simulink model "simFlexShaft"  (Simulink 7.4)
settings: Solver=ode45  StartTime=0.0  StopTime=inf  RelTol=1e-3
InitFcn:
  | updateVarParamFlexShaft
StopFcn:
  | stopFcnFlexShaft
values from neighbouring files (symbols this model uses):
  cmd = 0    [initFcnFlexShaft.m]    (also in updateVarParamFlexShaft.m = 1)
  controllerSel = 0    [initFcnFlexShaft.m]    (also in updateVarParamFlexShaft.m)
  denzTfLoopShapingController = [1 1e-3*ones(1,3)]    [initFcnFlexShaft.m]    (also in updateVarParamFlexShaft.m = Grd.den{1,1})
  fcnSel = 0    [initFcnFlexShaft.m]    (also in updateVarParamFlexShaft.m = 2)
  feedbackGainObserver = 1e-3*ones(N,1)    [initFcnFlexShaft.m]    (also in updateVarParamFlexShaft.m = L)
  feedbackGainStateController = 1e-3*ones(1,N)    [initFcnFlexShaft.m]    (also in updateVarParamFlexShaft.m = K_bar(1,2:end))
  integralGainPidController = 0.0    (= 0)    [initFcnFlexShaft.m]    (also in updateVarParamFlexShaft.m)
  integralGainStateController = 0.0    (= 0)    [initFcnFlexShaft.m]    (also in updateVarParamFlexShaft.m = K_bar(1,1))
  numzTfLoopShapingController = 1e-3*ones(1,4)    [initFcnFlexShaft.m]    (also in updateVarParamFlexShaft.m = Grd.num{1,1})
  proportionalGainPidController = 0.0    (= 0)    [initFcnFlexShaft.m]    (also in updateVarParamFlexShaft.m)
  sysMatrixAcPlant = sysc.Ac    [initFcnFlexShaft.m]    (also in updateVarParamFlexShaft.m)
  sysMatrixAdObserver = sysd.a    [initFcnFlexShaft.m]    (also in updateVarParamFlexShaft.m = Ad)
  sysMatrixBcPlant = sysc.Bc    [initFcnFlexShaft.m]    (also in updateVarParamFlexShaft.m)
  sysMatrixBduObserver = sysd.b(:,1)    [initFcnFlexShaft.m]    (also in updateVarParamFlexShaft.m = Bd(:,1))
  sysMatrixCcPlant = sysc.Cc    [initFcnFlexShaft.m]    (also in updateVarParamFlexShaft.m)
  sysMatrixCdObserver = sysd.c    [initFcnFlexShaft.m]    (also in updateVarParamFlexShaft.m = Cd)
  sysMatrixDcPlant = sysc.Dc    [initFcnFlexShaft.m]    (also in updateVarParamFlexShaft.m)
undefined symbols (not defined in the file or in its folder): constParamFlexShaft
libraries: simulink x14, dspsnks4 x2, simulink_extras x1
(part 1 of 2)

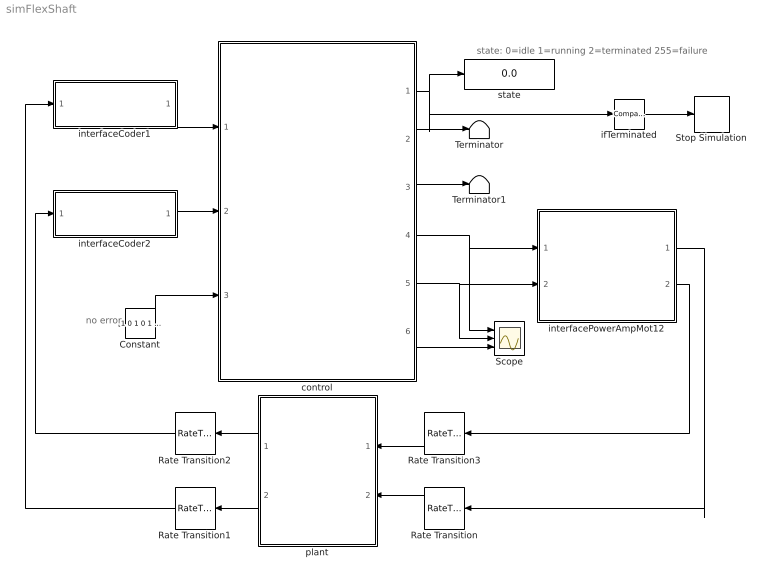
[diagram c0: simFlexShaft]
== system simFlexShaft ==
  note: state: 0=idle 1=running 2=terminated 255=failure
  note: no error
  Constant : Constant  Value=[1 0 1 0 1 0 0 0 0 0 0 0]
  Rate Transition{,1..3} (4 alike) : RateTransition
  Scope : Scope  NumInputPorts=3
  Stop Simulation : Stop
  Terminator : Terminator
  Terminator1 : Terminator
  control : Subsystem  TreatAsAtomicUnit=on  SystemSampleTime=constParamFlexShaft.samplingTime  mask{constParam=constParamFlexShaft.control, cmd=cmd, fcnSel=fcnSel, controllerSel=controllerSel, proportionalGainPidController=proportionalGainPidController, integralGainPidController=integralGainPidController, numzTfLoopShapingController=numzTfLoopShapingController, denzTfLoopShapingController=denzTfLoopShapingController, integralGainStateController=integralGainStateController, feedbackGainStateController=feedbackGainStateController, sysMatrixAdObserver=sysMatrixAdObserver, sysMatrixBduObserver=sysMatrixBduObserver, sysMatrixCdObserver=sysMatrixCdObserver, feedbackGainObserver=feedbackGainObserver}
      mask prompts: constParam "Constant:"; cmd "Command:"; fcnSel "Function Selector:"; controllerSel "Controller Selector:"; proportionalGainPidController "Proportional Gain PID Controller:"; integralGainPidController "Integral Gain PID Controller:"; numzTfLoopShapingController "Numerator Transfer Function Loop Shaping Controller:"; denzTfLoopShapingController "Denumerator Transfer Function Loop Shaping Controller"; integralGainStateController "Integral Gain State Controller:"; feedbackGainStateController "Feedback Gain State Controller"; sysMatrixAdObserver "System Matrix Ad Observer:"; sysMatrixBduObserver "System Matrix Bdu Observer:"; sysMatrixCdObserver "System Matrix Cd Observer:"; feedbackGainObserver "Feedback Gain Observer:"
  ifTerminated : simulink/Logic and Bit Operations/Compare To Constant  SystemSampleTime=-1  relop===  const=2  LogicOutDataTypeMode=boolean
  interfaceCoder1 : Subsystem  mask{constParam=constParamFlexShaft.interfaceCoder1}
      mask prompts: constParam "Constant:"
  interfaceCoder2 : Subsystem  mask{constParam=constParamFlexShaft.interfaceCoder1}
      mask prompts: constParam "Constant:"
  interfacePowerAmpMot12 : Subsystem  mask{constParam=constParamFlexShaft.interfacePowerAmpMot12}
      mask prompts: constParam "Constant:"
  plant : Subsystem  mask{Ac=sysMatrixAcPlant, Bc=sysMatrixBcPlant, Cc=sysMatrixCcPlant, Dc=sysMatrixDcPlant}
      mask prompts: Ac "System Matrix A Plant:"; Bc "System Matrix B Plant:"; Cc "System Matrix C Plant:"; Dc "System Matrix D Plant:"
  state : Display
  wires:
  control/4(refVoltageMot1) -> interfacePowerAmpMot12/1(refVoltageMot1), Scope/1
  control/5(refCurrentMot2) -> interfacePowerAmpMot12/2(refCurrentMot2), Scope/2
  control/6(estimatedVelMot1) -> Scope/3
  control/1(state) -> state/1, ifTerminated/1
  control/2(errorID) -> Terminator/1
  control/3(reset) -> Terminator1/1
  Rate Transition/1 -> plant/2(voltageMot1)
  plant/2(posMot1) -> Rate Transition1/1
  plant/1(posMot2) -> Rate Transition2/1
  Rate Transition3/1 -> plant/1(currentMot2)
  interfacePowerAmpMot12/2(currentMot2) -> Rate Transition3/1
  interfacePowerAmpMot12/1(voltageMot1) -> Rate Transition/1
  Rate Transition2/1 -> interfaceCoder2/1(posMot)
  Rate Transition1/1 -> interfaceCoder1/1(posMot)
  interfaceCoder1/1(deltaPosMot) -> control/1(deltaPosMot1)
  interfaceCoder2/1(deltaPosMot) -> control/2(deltaPosMot2)
  Constant/1 -> control/3(errorVector)
  ifTerminated/1 -> Stop Simulation/1

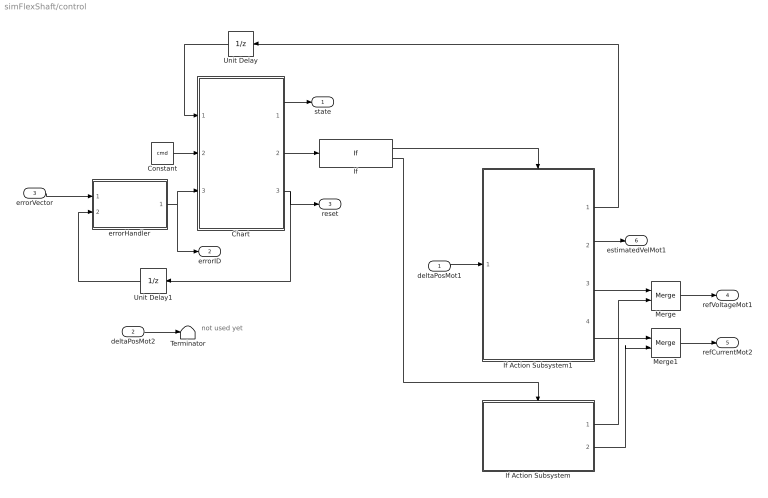
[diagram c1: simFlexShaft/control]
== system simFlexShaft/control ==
  note: not used yet
  deltaPosMot1 : Inport
  deltaPosMot2 : Inport  Port=2
  errorVector : Inport  Port=3
  Chart : Stateflow chart  TreatAsAtomicUnit=on
  Constant : Constant  Value=cmd  OutDataTypeMode=uint8  OutDataTypeStr=uint8  SampleTime=-1
  If : If  IfExpression=u1 == 1
  If Action Subsystem : Subsystem  TreatAsAtomicUnit=on
  If Action Subsystem1 : Subsystem  TreatAsAtomicUnit=on
  Merge : Merge  InitialOutput=0.0
  Merge1 : Merge  InitialOutput=0.0
  Terminator : Terminator
  Unit Delay : UnitDelay  SampleTime=-1
  Unit Delay1 : UnitDelay  SampleTime=-1
  errorHandler : Subsystem  TreatAsAtomicUnit=on
  state : Outport
  errorID : Outport  Port=2
  reset : Outport  Port=3
  refVoltageMot1 : Outport  Port=4
  refCurrentMot2 : Outport  Port=5
  estimatedVelMot1 : Outport  Port=6
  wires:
  Chart/1(state) -> state/1
  If/2 -> If Action Subsystem/Action
  If/1 -> If Action Subsystem1/Action
  If Action Subsystem1/3(refVoltageMot1) -> Merge/1
  If Action Subsystem1/4(refCurrentMot2) -> Merge1/1
  If Action Subsystem/1(refVoltageMot1) -> Merge/2
  If Action Subsystem/2(refCurrentMot2) -> Merge1/2
  Merge/1 -> refVoltageMot1/1
  Merge1/1 -> refCurrentMot2/1
  deltaPosMot2/1 -> Terminator/1
  Chart/2(enable) -> If/1
  Chart/3(reset) -> reset/1, Unit Delay1/1
  errorHandler/1(errorID) -> errorID/1, Chart/3(errorID)
  Unit Delay1/1 -> errorHandler/2(reset)
  Unit Delay/1 -> Chart/1(fcnState)
  If Action Subsystem1/1(fcnState) -> Unit Delay/1
  deltaPosMot1/1 -> If Action Subsystem1/1(deltaPosMot1)
  If Action Subsystem1/2(estimatedVelMot1) -> estimatedVelMot1/1
  errorVector/1 -> errorHandler/1(errorVector)
  Constant/1 -> Chart/2(cmd)

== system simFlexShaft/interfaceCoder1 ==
  posMot : Inport
  Quantizer : Quantizer  QuantizationInterval=constParam.resolution
  Sum : Sum  Inputs=|+-
  Unit Delay : UnitDelay  SampleTime=-1
  deltaPosMot : Outport
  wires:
  Quantizer/1 -> Sum/1, Unit Delay/1
  Unit Delay/1 -> Sum/2
  posMot/1 -> Quantizer/1
  Sum/1 -> deltaPosMot/1

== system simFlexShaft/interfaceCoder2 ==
  posMot : Inport
  Quantizer : Quantizer  QuantizationInterval=constParam.resolution
  Sum : Sum  Inputs=|+-
  Unit Delay : UnitDelay  SampleTime=-1
  deltaPosMot : Outport
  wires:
  Quantizer/1 -> Sum/1, Unit Delay/1
  Unit Delay/1 -> Sum/2
  posMot/1 -> Quantizer/1
  Sum/1 -> deltaPosMot/1

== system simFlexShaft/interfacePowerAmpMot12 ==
  refVoltageMot1 : Inport
  refCurrentMot2 : Inport  Port=2
  Quantizer : Quantizer  QuantizationInterval=constParam.voltageResolution
  Quantizer1 : Quantizer  QuantizationInterval=constParam.currentResolution
  Saturation : Saturate  UpperLimit=constParam.maxVoltageMot1  LowerLimit=-constParam.maxVoltageMot1
  Saturation1 : Saturate  UpperLimit=constParam.maxCurrentMot2  LowerLimit=-constParam.maxCurrentMot2
  voltageMot1 : Outport
  currentMot2 : Outport  Port=2
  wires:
  Quantizer/1 -> voltageMot1/1
  refVoltageMot1/1 -> Saturation/1
  refCurrentMot2/1 -> Saturation1/1
  Saturation/1 -> Quantizer/1
  Saturation1/1 -> Quantizer1/1
  Quantizer1/1 -> currentMot2/1

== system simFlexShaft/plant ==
  note: velMot1
  note: velMot2
  note: currentMot1
  currentMot2 : Inport
  voltageMot1 : Inport  Port=2
  Demux1 : Demux  Outputs=5
  Mux : Mux  Inputs=2
  State-Space : StateSpace  A=Ac  B=Bc  C=Cc  D=Dc  X0=0.0
  Terminator : Terminator
  Terminator1 : Terminator
  Terminator2 : Terminator
  posMot2 : Outport
  posMot1 : Outport  Port=2
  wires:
  State-Space/1 -> Demux1/1
  Mux/1 -> State-Space/1
  voltageMot1/1 -> Mux/1
  currentMot2/1 -> Mux/2
  Demux1/4 -> posMot2/1
  Demux1/3 -> posMot1/1
  Demux1/1 -> Terminator/1
  Demux1/2 -> Terminator1/1
  Demux1/5 -> Terminator2/1

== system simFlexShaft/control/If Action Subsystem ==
  Action Port : ActionPort  InitializeStates=reset  ActionType=else
  Constant : Constant  Value=0.0
  Gain : Gain
  Gain1 : Gain
  refVoltageMot1 : Outport  InitialOutput=0.0
  refCurrentMot2 : Outport  Port=2  InitialOutput=0.0
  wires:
  Gain/1 -> refVoltageMot1/1
  Gain1/1 -> refCurrentMot2/1
  Constant/1 -> Gain/1, Gain1/1

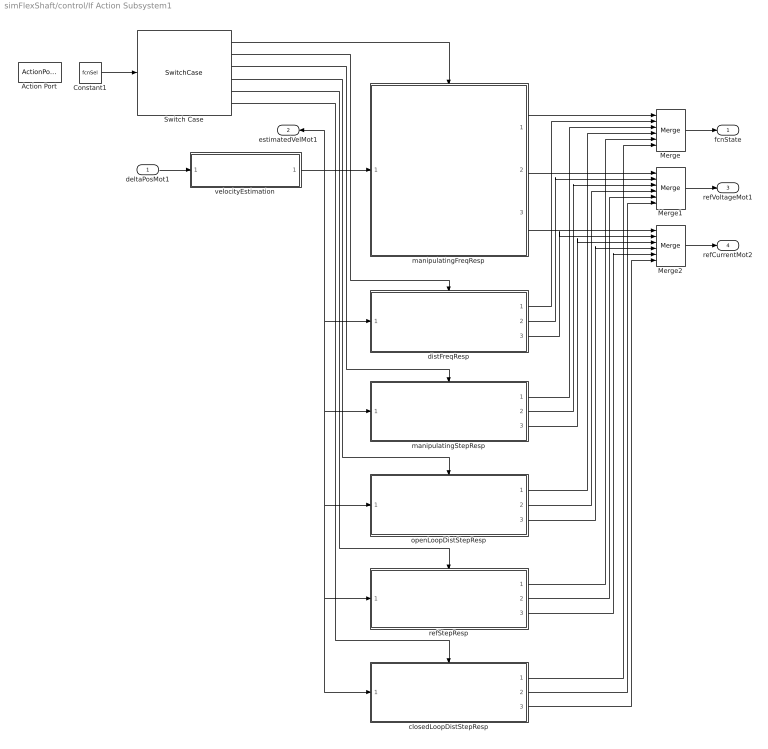
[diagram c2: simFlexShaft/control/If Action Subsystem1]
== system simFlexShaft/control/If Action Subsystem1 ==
  deltaPosMot1 : Inport
  Action Port : ActionPort  InitializeStates=reset  ActionType=then
  Constant1 : Constant  Value=fcnSel  OutDataTypeMode=uint8  OutDataTypeStr=uint8  SampleTime=-1
  Merge : Merge  Inputs=6
  Merge1 : Merge  Inputs=6
  Merge2 : Merge  Inputs=6
  Switch Case : SwitchCase  CaseConditions={0,1,2,3,4,5}  ShowDefaultCase=off
  closedLoopDistStepResp : Subsystem  TreatAsAtomicUnit=on  mask{constParam=constParam.closedLoopDistStepResp, controllerSel=controllerSel, proportionalGainPidController=proportionalGainPidController, integralGainPidController=integralGainPidController, numzTfLoopShapingController=numzTfLoopShapingController, denzTfLoopShapingController=denzTfLoopShapingController, integralGainStateController=integralGainStateController, feedbackGainStateController=feedbackGainStateController, sysMatrixAdObserver=sysMatrixAdObserver, sysMatrixBduObserver=sysMatrixBduObserver, sysMatrixCdObserver=sysMatrixCdObserver, feedbackGainObserver=feedbackGainObserver}
      mask prompts: constParam "Constant:"; controllerSel "Controller Selector:"; proportionalGainPidController "Proportional Gain PID Controller:"; integralGainPidController "Integral Gain PI Controller:"; numzTfLoopShapingController "Numerator Transfer Function Loop Shaping Controller:"; denzTfLoopShapingController "Denumerator Transfer Function Loop Shaping Controller."; integralGainStateController "Integral Gain State Controller:"; feedbackGainStateController "Feedback Gain State Controller."; sysMatrixAdObserver "System Matrix Ad Observer:"; sysMatrixBduObserver "System Matrix Bdu Observer:"; sysMatrixCdObserver "System Matrix Cd Observer:"; feedbackGainObserver "Feedback Gain Observer:"
  distFreqResp : Subsystem  TreatAsAtomicUnit=on  mask{constParam=constParam.distFreqResp}
      mask prompts: constParam "Constant:"
  manipulatingFreqResp : Subsystem  TreatAsAtomicUnit=on  mask{constParam=constParam.manipulatingFreqResp}
      mask prompts: constParam "Constant:"
  manipulatingStepResp : Subsystem  TreatAsAtomicUnit=on  mask{constParam=constParam.manipulatingStepResp}
      mask prompts: constParam "Constant:"
  openLoopDistStepResp : Subsystem  TreatAsAtomicUnit=on  mask{constParam=constParam.openLoopDistStepResp}
      mask prompts: constParam "Constant:"
  refStepResp : Subsystem  TreatAsAtomicUnit=on  mask{constParam=constParam.refStepResp, controllerSel=controllerSel, proportionalGainPidController=proportionalGainPidController, integralGainPidController=integralGainPidController, numzTfLoopShapingController=numzTfLoopShapingController, denzTfLoopShapingController=denzTfLoopShapingController, integralGainStateController=integralGainStateController, feedbackGainStateController=feedbackGainStateController, sysMatrixAdObserver=sysMatrixAdObserver, sysMatrixBduObserver=sysMatrixBduObserver, sysMatrixCdObserver=sysMatrixCdObserver, feedbackGainObserver=feedbackGainObserver}
      mask prompts: constParam "Constant:"; controllerSel "Controller Selector:"; proportionalGainPidController "Proportional Gain PID Controller:"; integralGainPidController "Integral Gain PID Controller:"; numzTfLoopShapingController "Numerator Transfer Function Loop Shaping Controller:"; denzTfLoopShapingController "Denumerator Transfer Function Loop Shaping Controller."; integralGainStateController "Integral Gain State Controller:"; feedbackGainStateController "Feedback Gain State Controller."; sysMatrixAdObserver "System Matrix Ad Observer:"; sysMatrixBduObserver "System Matrix Bdu Observer:"; sysMatrixCdObserver "System Matrix Cd Observer:"; feedbackGainObserver "Feedback Gain Observer:"
  velocityEstimation : Subsystem  TreatAsAtomicUnit=on  mask{constParam=constParam.velEstimation}
      mask prompts: constParam "Constant:"
  fcnState : Outport  InitialOutput=0
  estimatedVelMot1 : Outport  Port=2  InitialOutput=0
  refVoltageMot1 : Outport  Port=3  InitialOutput=0.0
  refCurrentMot2 : Outport  Port=4  InitialOutput=0.0
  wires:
  deltaPosMot1/1 -> velocityEstimation/1(deltaPosMot1)
  Switch Case/1 -> manipulatingFreqResp/Action
  velocityEstimation/1(estimatedVelMot1) -> estimatedVelMot1/1, distFreqResp/1(estimatedVelMot1), refStepResp/1(estimatedVelMot1), closedLoopDistStepResp/1(estimatedVelMot1), openLoopDistStepResp/1(estimatedVelMot1), manipulatingStepResp/1(estimatedVelMot1), manipulatingFreqResp/1(estimatedVelMot1)
  Merge/1 -> fcnState/1
  Switch Case/2 -> distFreqResp/Action
  distFreqResp/1(fcnState) -> Merge/2
  Merge1/1 -> refVoltageMot1/1
  Merge2/1 -> refCurrentMot2/1
  distFreqResp/2(refVoltageMot1) -> Merge1/2
  distFreqResp/3(refCurrentMot2) -> Merge2/2
  Switch Case/3 -> manipulatingStepResp/Action
  manipulatingStepResp/1(fcnState) -> Merge/3
  manipulatingStepResp/2(refVoltageMot1) -> Merge1/3
  manipulatingStepResp/3(refCurrentMot2) -> Merge2/3
  Switch Case/4 -> openLoopDistStepResp/Action
  Switch Case/5 -> refStepResp/Action
  Switch Case/6 -> closedLoopDistStepResp/Action
  openLoopDistStepResp/1(fcnState) -> Merge/4
  closedLoopDistStepResp/1(fcnState) -> Merge/6
  openLoopDistStepResp/2(refVoltageMot1) -> Merge1/4
  refStepResp/3(refCurrentMot2) -> Merge2/5
  closedLoopDistStepResp/2(refVoltageMot1) -> Merge1/6
  closedLoopDistStepResp/3(refCurrentMot2) -> Merge2/6
  openLoopDistStepResp/3(refCurrentMot2) -> Merge2/4
  refStepResp/1(fcnState) -> Merge/5
  refStepResp/2(refVoltageMot1) -> Merge1/5
  manipulatingFreqResp/1(fcnState) -> Merge/1
  manipulatingFreqResp/2(refVoltageMot1) -> Merge1/1
  manipulatingFreqResp/3(refCurrentMot2) -> Merge2/1
  Constant1/1 -> Switch Case/1

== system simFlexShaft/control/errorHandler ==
  note: caution!!! errors from coder 2 are not analyzed yet
  note: error latch
  errorVector : Inport
  reset : Inport  Port=2
  Compare To Zero : simulink/Logic and Bit Operations/Compare To Zero  SystemSampleTime=-1  relop=>  LogicOutDataTypeMode=boolean
  Data Type Conversion : DataTypeConversion  OutDataTypeMode=uint8  OutDataTypeStr=uint8
  Detect Rise Positive : simulink/Logic and Bit Operations/Detect Rise Positive  SystemSampleTime=-1  vinit=0
  S-R Flip-Flop : simulink_extras/Flip Flops/S-R Flip-Flop  SystemSampleTime=-1  initial_condition=0
  Switch : Switch  Criteria=u2 > Threshold  OutDataTypeStr=Inherit: Inherit via back propagation
  Terminator : Terminator
  Truth Table : Stateflow chart  TreatAsAtomicUnit=on
  Unit Delay Resettable : simulink/Additional Math & Discrete/Additional Discrete/Unit Delay Resettable  SystemSampleTime=-1  vinit=0  tsamp=-1
  errorID : Outport
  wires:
  Truth Table/1(errorID) -> Compare To Zero/1, Switch/1
  errorVector/1 -> Truth Table/1(errorVector)
  S-R Flip-Flop/2 -> Terminator/1
  S-R Flip-Flop/1 -> Detect Rise Positive/1
  reset/1 -> S-R Flip-Flop/2, Unit Delay Resettable/2
  Compare To Zero/1 -> S-R Flip-Flop/1
  Detect Rise Positive/1 -> Switch/2
  Switch/1 -> Unit Delay Resettable/1
  Unit Delay Resettable/1 -> Switch/3, Data Type Conversion/1
  Data Type Conversion/1 -> errorID/1

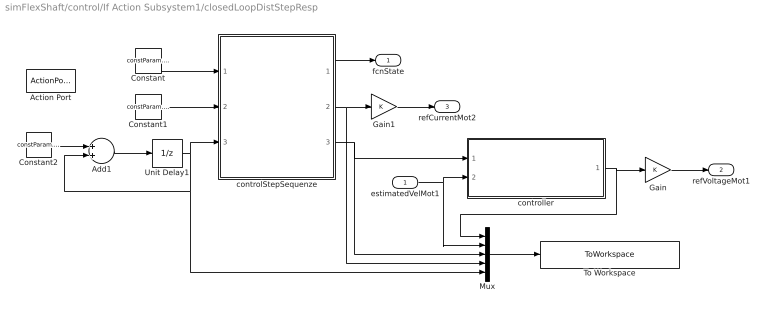
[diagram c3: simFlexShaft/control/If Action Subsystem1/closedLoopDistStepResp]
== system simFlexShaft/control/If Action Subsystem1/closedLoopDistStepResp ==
  estimatedVelMot1 : Inport
  Action Port : ActionPort  InitializeStates=reset  ActionType=case
  Add1 : Sum
  Constant : Constant  Value=constParam.nrOfSteps  OutDataTypeMode=uint8  OutDataTypeStr=uint8
  Constant1 : Constant  Value=constParam.stepSequenze  OutDataTypeMode=double  OutDataTypeStr=double
  Constant2 : Constant  Value=constParam.samplingTime  OutDataTypeMode=double  OutDataTypeStr=double
  Gain : Gain
  Gain1 : Gain
  Mux : Mux  Inputs=5
  To Workspace : ToWorkspace  VariableName=recDataClosedLoopDistStepResp  SampleTime=-1  SaveFormat=Array
  Unit Delay1 : UnitDelay  X0=0.0  SampleTime=-1
  controlStepSequenze : Stateflow chart  TreatAsAtomicUnit=on
  controller : Subsystem  mask{constParam=constParam.feedbackController, controllerSel=controllerSel, proportionalGainPidController=proportionalGainPidController, integralGainPidController=integralGainPidController, numzTfLoopShapingController=numzTfLoopShapingController, denzTfLoopShapingController=denzTfLoopShapingController, integralGainStateController=integralGainStateController, feedbackGainStateController=feedbackGainStateController, sysMatrixAdObserver=sysMatrixAdObserver, sysMatrixBduObserver=sysMatrixBduObserver, sysMatrixCdObserver=sysMatrixCdObserver, feedbackGainObserver=feedbackGainObserver}
      mask prompts: constParam "Constant:"; controllerSel "Controller Selector:"; proportionalGainPidController "Proportional Gain PID Controller:"; integralGainPidController "Integral Gain PI Controller:"; numzTfLoopShapingController "Numerator Transfer Function Loop Shaping Controller:"; denzTfLoopShapingController "Denumerator Transfer Function Loop Shaping Controller:"; integralGainStateController "Integral Gain State Controller:"; feedbackGainStateController "Feedback Gain State Controller:"; sysMatrixAdObserver "System Matrix Ad Observer:"; sysMatrixBduObserver "System Matrix Bdu Observer:"; sysMatrixCdObserver "System Matrix Cd Observer:"; feedbackGainObserver "Feedback Gain Oberver:"
  fcnState : Outport  InitialOutput=0
  refVoltageMot1 : Outport  Port=2  InitialOutput=0.0
  refCurrentMot2 : Outport  Port=3  InitialOutput=0.0
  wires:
  controlStepSequenze/1(fcnState) -> fcnState/1
  Constant1/1 -> controlStepSequenze/2(stepSeq)
  Constant/1 -> controlStepSequenze/1(nrOfSteps)
  Mux/1 -> To Workspace/1
  Gain/1 -> refVoltageMot1/1
  Gain1/1 -> refCurrentMot2/1
  controlStepSequenze/2(stepVal1) -> Gain1/1, Mux/4
  Unit Delay1/1 -> controlStepSequenze/3(time), Add1/2, Mux/5
  Add1/1 -> Unit Delay1/1
  Constant2/1 -> Add1/1
  controller/1(refVoltagMot1) -> Gain/1, Mux/1
  estimatedVelMot1/1 -> Mux/2, controller/2(estimatedVelMot1)
  controlStepSequenze/3(stepVal2) -> Mux/3, controller/1(refVelMot1)

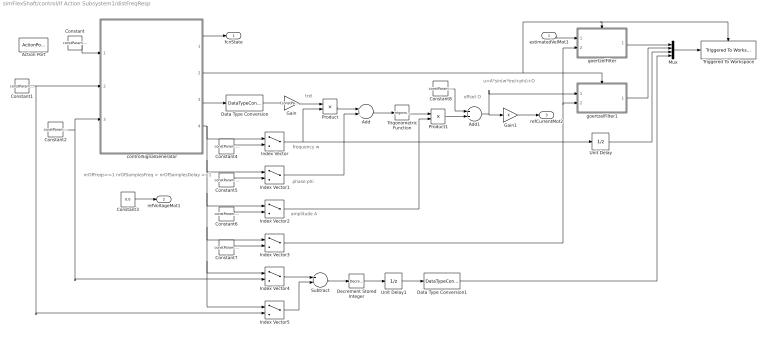
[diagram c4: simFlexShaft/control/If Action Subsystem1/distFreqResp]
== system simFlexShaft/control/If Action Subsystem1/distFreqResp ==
  note: frequency w
  note: phase phi
  note: amplitude A
  note: nrOfFreqs>=1 nrOfSamplesFreq > nrOfSamplesDelay >=1
  note: offset O
  note: trel
  note: u=A*sin(w*trel+phi)+O
  estimatedVelMot1 : Inport
  Action Port : ActionPort  InitializeStates=reset  ActionType=case
  Add : Sum
  Add1 : Sum
  Constant : Constant  Value=constParam.nrOfFreqs  VectorParams1D=off  OutDataTypeMode=uint8  OutDataTypeStr=uint8
  Constant1 : Constant  Value=constParam.nrOfSamplesDelay  VectorParams1D=off  OutDataTypeMode=uint32  OutDataTypeStr=uint32
  Constant2 : Constant  Value=constParam.nrOfSamplesFreq  VectorParams1D=off  OutDataTypeMode=uint32  OutDataTypeStr=uint32
  Constant3 : Constant  Value=0.0
  Constant4 : Constant  Value=constParam.freqs
  Constant5 : Constant  Value=constParam.phases
  Constant6 : Constant  Value=constParam.amplitudes
  Constant7 : Constant  Value=constParam.filterCoeffs
  Constant8 : Constant  Value=constParam.offset
  Data Type Conversion : DataTypeConversion  OutDataTypeMode=double  OutDataTypeStr=double
  Data Type Conversion1 : DataTypeConversion  OutDataTypeMode=double  OutDataTypeStr=double
  Decrement Stored Integer : simulink/Additional Math & Discrete/Additional Math: Increment - Decrement/Decrement Stored Integer  SystemSampleTime=-1
  Gain : Gain  Gain=constParam.samplingTime
  Gain1 : Gain
  Index Vector{,1..5} (6 alike) : MultiPortSwitch  Inputs=1
  Mux : Mux
  Product : Product
  Product1 : Product
  Subtract : Sum  Inputs=+-
  Triggered To Workspace : dspsnks4/Triggered To Workspace  SystemSampleTime=-1  TriggerType=Falling edge  VariableName=recDataDistFreqResp  Buffer=1000
  Trigonometric Function : Trigonometry
  Unit Delay : UnitDelay  X0=constParam.freqs(1,1)  SampleTime=-1
  Unit Delay1 : UnitDelay  X0=(constParam.nrOfSamplesFreq(1,1)-constParam.nrOfSamplesDelay(1,1))  SampleTime=-1
  controlSignalGenerator : Stateflow chart  TreatAsAtomicUnit=on
  goertzelFilter : Subsystem  TreatAsAtomicUnit=on
  goertzelFilter1 : Subsystem  TreatAsAtomicUnit=on
  fcnState : Outport  InitialOutput=0
  refVoltageMot1 : Outport  Port=2  InitialOutput=0.0
  refCurrentMot2 : Outport  Port=3  InitialOutput=0.0
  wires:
  Constant3/1 -> refVoltageMot1/1
  Data Type Conversion/1 -> Gain/1
  Constant4/1 -> Index Vector/2
  Constant5/1 -> Index Vector1/2
  Constant6/1 -> Index Vector2/2
  Constant/1 -> controlSignalGenerator/1(nrOfFreqs)
  Constant1/1 -> Index Vector5/2, controlSignalGenerator/2(nrOfSamplesDelay)
  Constant2/1 -> Index Vector4/2, controlSignalGenerator/3(nrOfSamplesFreq)
  controlSignalGenerator/1(fcnState) -> fcnState/1
  Add1/1 -> Gain1/1, goertzelFilter1/1(xk)
  Constant7/1 -> Index Vector3/2
  goertzelFilter/1(vk) -> Mux/1
  goertzelFilter1/1(vk) -> Mux/2
  Mux/1 -> Triggered To Workspace/1
  Index Vector4/1 -> Subtract/1
  Index Vector5/1 -> Subtract/2
  Subtract/1 -> Decrement Stored Integer/1
  Decrement Stored Integer/1 -> Unit Delay1/1
  Add/1 -> Trigonometric Function/1
  Unit Delay1/1 -> Data Type Conversion1/1
  Unit Delay/1 -> Mux/3
  Product1/1 -> Add1/2
  Constant8/1 -> Add1/1
  Gain/1 -> Product/1
  Product/1 -> Add/1
  Trigonometric Function/1 -> Product1/1
  Index Vector/1 -> Product/2, Unit Delay/1
  Index Vector1/1 -> Add/2
  Index Vector2/1 -> Product1/2
  controlSignalGenerator/3(krel) -> Data Type Conversion/1
  controlSignalGenerator/4(idx) -> Index Vector/1, Index Vector1/1, Index Vector2/1, Index Vector4/1, Index Vector5/1, Index Vector3/1
  Gain1/1 -> refCurrentMot2/1
  Index Vector3/1 -> goertzelFilter1/2(ak), goertzelFilter/2(ak)
  estimatedVelMot1/1 -> goertzelFilter/1(xk)
  controlSignalGenerator/2(enFilter) -> goertzelFilter1/Enable, goertzelFilter/Enable, Triggered To Workspace/Trigger
  Data Type Conversion1/1 -> Mux/4

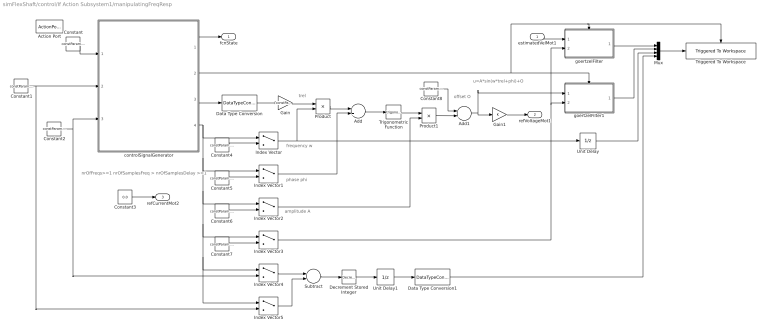
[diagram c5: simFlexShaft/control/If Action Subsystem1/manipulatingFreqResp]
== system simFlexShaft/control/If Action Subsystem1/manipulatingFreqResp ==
  note: frequency w
  note: phase phi
  note: amplitude A
  note: nrOfFreqs>=1 nrOfSamplesFreq > nrOfSamplesDelay >=1
  note: offset O
  note: trel
  note: u=A*sin(w*trel+phi)+O
  estimatedVelMot1 : Inport
  Action Port : ActionPort  InitializeStates=reset  ActionType=case
  Add : Sum
  Add1 : Sum
  Constant : Constant  Value=constParam.nrOfFreqs*1  VectorParams1D=off  OutDataTypeMode=uint8  OutDataTypeStr=uint8
  Constant1 : Constant  Value=constParam.nrOfSamplesDelay.*1  VectorParams1D=off  OutDataTypeMode=uint32  OutDataTypeStr=uint32
  Constant2 : Constant  Value=constParam.nrOfSamplesFreq.*1  VectorParams1D=off  OutDataTypeMode=uint32  OutDataTypeStr=uint32
  Constant3 : Constant  Value=0.0
  Constant4 : Constant  Value=constParam.freqs.*1
  Constant5 : Constant  Value=constParam.phases.*1
  Constant6 : Constant  Value=constParam.amplitudes.*1
  Constant7 : Constant  Value=constParam.filterCoeffs.*1
  Constant8 : Constant  Value=constParam.offset*1
  Data Type Conversion : DataTypeConversion  OutDataTypeMode=double  OutDataTypeStr=double
  Data Type Conversion1 : DataTypeConversion  OutDataTypeMode=double  OutDataTypeStr=double
  Decrement Stored Integer : simulink/Additional Math & Discrete/Additional Math: Increment - Decrement/Decrement Stored Integer  SystemSampleTime=-1
  Gain : Gain  Gain=constParam.samplingTime*1
  Gain1 : Gain
  Index Vector{,1..5} (6 alike) : MultiPortSwitch  Inputs=1
  Mux : Mux
  Product : Product
  Product1 : Product
  Subtract : Sum  Inputs=+-
  Triggered To Workspace : dspsnks4/Triggered To Workspace  SystemSampleTime=-1  TriggerType=Falling edge  VariableName=recDataManipulatingFreqResp  Buffer=1000
  Trigonometric Function : Trigonometry
  Unit Delay : UnitDelay  X0=constParam.freqs(1,1)*1  SampleTime=-1
  Unit Delay1 : UnitDelay  X0=(constParam.nrOfSamplesFreq(1,1)-constParam.nrOfSamplesDelay(1,1))*1  SampleTime=-1
  controlSignalGenerator : Stateflow chart  TreatAsAtomicUnit=on
  goertzelFilter : Subsystem  TreatAsAtomicUnit=on
  goertzelFilter1 : Subsystem  TreatAsAtomicUnit=on
  fcnState : Outport  InitialOutput=0
  refVoltageMot1 : Outport  Port=2  InitialOutput=0.0
  refCurrentMot2 : Outport  Port=3  InitialOutput=0.0
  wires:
  Data Type Conversion/1 -> Gain/1
  Constant4/1 -> Index Vector/2
  Constant5/1 -> Index Vector1/2
  Constant6/1 -> Index Vector2/2
  Constant/1 -> controlSignalGenerator/1(nrOfFreqs)
  Constant1/1 -> Index Vector5/2, controlSignalGenerator/2(nrOfSamplesDelay)
  Constant2/1 -> Index Vector4/2, controlSignalGenerator/3(nrOfSamplesFreq)
  controlSignalGenerator/1(fcnState) -> fcnState/1
  Add1/1 -> Gain1/1, goertzelFilter1/1(xk)
  Constant7/1 -> Index Vector3/2
  goertzelFilter/1(vk) -> Mux/1
  goertzelFilter1/1(vk) -> Mux/2
  Mux/1 -> Triggered To Workspace/1
  Index Vector4/1 -> Subtract/1
  Index Vector5/1 -> Subtract/2
  Subtract/1 -> Decrement Stored Integer/1
  Decrement Stored Integer/1 -> Unit Delay1/1
  Add/1 -> Trigonometric Function/1
  Unit Delay1/1 -> Data Type Conversion1/1
  Unit Delay/1 -> Mux/3
  Product1/1 -> Add1/2
  Constant8/1 -> Add1/1
  Gain/1 -> Product/1
  Product/1 -> Add/1
  Trigonometric Function/1 -> Product1/1
  Index Vector/1 -> Product/2, Unit Delay/1
  Index Vector1/1 -> Add/2
  Index Vector2/1 -> Product1/2
  controlSignalGenerator/3(krel) -> Data Type Conversion/1
  controlSignalGenerator/4(idx) -> Index Vector/1, Index Vector1/1, Index Vector2/1, Index Vector4/1, Index Vector5/1, Index Vector3/1
  Index Vector3/1 -> goertzelFilter1/2(ak), goertzelFilter/2(ak)
  estimatedVelMot1/1 -> goertzelFilter/1(xk)
  controlSignalGenerator/2(enFilter) -> goertzelFilter1/Enable, goertzelFilter/Enable, Triggered To Workspace/Trigger
  Data Type Conversion1/1 -> Mux/4
  Constant3/1 -> refCurrentMot2/1
  Gain1/1 -> refVoltageMot1/1

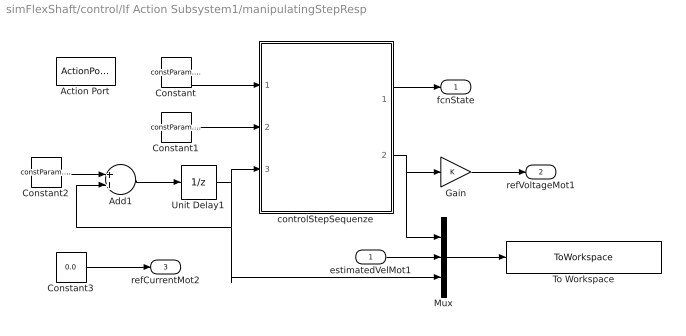
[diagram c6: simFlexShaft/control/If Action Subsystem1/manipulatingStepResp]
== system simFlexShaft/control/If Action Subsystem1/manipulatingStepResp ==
  estimatedVelMot1 : Inport
  Action Port : ActionPort  InitializeStates=reset  ActionType=case
  Add1 : Sum
  Constant : Constant  Value=constParam.nrOfSteps  OutDataTypeMode=uint8  OutDataTypeStr=uint8
  Constant1 : Constant  Value=constParam.stepSequenze  OutDataTypeMode=double  OutDataTypeStr=double
  Constant2 : Constant  Value=constParam.samplingTime  OutDataTypeMode=double  OutDataTypeStr=double
  Constant3 : Constant  Value=0.0
  Gain : Gain
  Mux : Mux  Inputs=3
  To Workspace : ToWorkspace  VariableName=recDataManipulatingStepResp  SampleTime=-1  SaveFormat=Array
  Unit Delay1 : UnitDelay  X0=0.0  SampleTime=-1
  controlStepSequenze : Stateflow chart  TreatAsAtomicUnit=on
  fcnState : Outport  InitialOutput=0
  refVoltageMot1 : Outport  Port=2  InitialOutput=0.0
  refCurrentMot2 : Outport  Port=3  InitialOutput=0.0
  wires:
  Constant3/1 -> refCurrentMot2/1
  Gain/1 -> refVoltageMot1/1
  Unit Delay1/1 -> controlStepSequenze/3(time), Add1/2, Mux/3
  Add1/1 -> Unit Delay1/1
  Constant2/1 -> Add1/1
  controlStepSequenze/1(fcnState) -> fcnState/1
  controlStepSequenze/2(stepVal) -> Gain/1, Mux/1
  Constant/1 -> controlStepSequenze/1(nrOfSteps)
  Constant1/1 -> controlStepSequenze/2(stepSeq)
  Mux/1 -> To Workspace/1
  estimatedVelMot1/1 -> Mux/2

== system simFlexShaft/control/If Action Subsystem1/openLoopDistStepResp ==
  estimatedVelMot1 : Inport
  Action Port : ActionPort  InitializeStates=reset  ActionType=case
  Add1 : Sum
  Constant : Constant  Value=constParam.nrOfSteps  OutDataTypeMode=uint8  OutDataTypeStr=uint8
  Constant1 : Constant  Value=constParam.stepSequenze  OutDataTypeMode=double  OutDataTypeStr=double
  Constant2 : Constant  Value=constParam.samplingTime  OutDataTypeMode=double  OutDataTypeStr=double
  Constant3 : Constant  Value=0.0
  Gain : Gain
  Mux : Mux  Inputs=3
  To Workspace : ToWorkspace  VariableName=recDataOpenLoopDistStepResp  SampleTime=-1  SaveFormat=Array
  Unit Delay1 : UnitDelay  X0=0.0  SampleTime=-1
  controlStepSequenze : Stateflow chart  TreatAsAtomicUnit=on
  fcnState : Outport  InitialOutput=0
  refVoltageMot1 : Outport  Port=2  InitialOutput=0.0
  refCurrentMot2 : Outport  Port=3  InitialOutput=0.0
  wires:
  Gain/1 -> refCurrentMot2/1
  Mux/1 -> To Workspace/1
  estimatedVelMot1/1 -> Mux/2
  Constant3/1 -> refVoltageMot1/1
  Unit Delay1/1 -> controlStepSequenze/3(time), Add1/2, Mux/3
  Add1/1 -> Unit Delay1/1
  Constant2/1 -> Add1/1
  Constant1/1 -> controlStepSequenze/2(stepSeq)
  Constant/1 -> controlStepSequenze/1(nrOfSteps)
  controlStepSequenze/2(stepVal) -> Gain/1, Mux/1
  controlStepSequenze/1(fcnState) -> fcnState/1

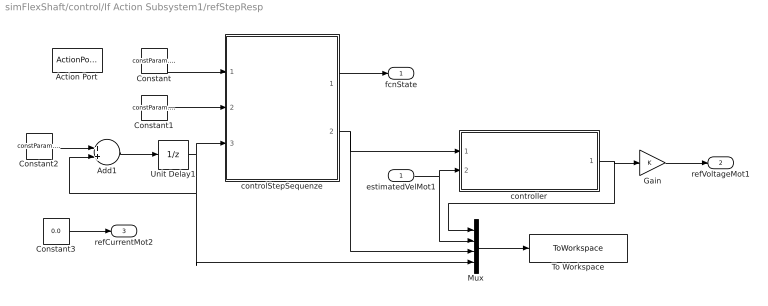
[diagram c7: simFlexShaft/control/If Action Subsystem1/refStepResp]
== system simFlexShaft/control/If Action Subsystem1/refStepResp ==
  estimatedVelMot1 : Inport
  Action Port : ActionPort  InitializeStates=reset  ActionType=case
  Add1 : Sum
  Constant : Constant  Value=constParam.nrOfSteps  OutDataTypeMode=uint8  OutDataTypeStr=uint8
  Constant1 : Constant  Value=constParam.stepSequenze  OutDataTypeMode=double  OutDataTypeStr=double
  Constant2 : Constant  Value=constParam.samplingTime  OutDataTypeMode=double  OutDataTypeStr=double
  Constant3 : Constant  Value=0.0
  Gain : Gain
  Mux : Mux
  To Workspace : ToWorkspace  VariableName=recDataRefStepResp  SampleTime=-1  SaveFormat=Array
  Unit Delay1 : UnitDelay  X0=0.0  SampleTime=-1
  controlStepSequenze : Stateflow chart  TreatAsAtomicUnit=on
  controller : Subsystem  mask{constParam=constParam.feedbackController, controllerSel=controllerSel, proportionalGainPidController=proportionalGainPidController, integralGainPidController=integralGainPidController, numzTfLoopShapingController=numzTfLoopShapingController, denzTfLoopShapingController=denzTfLoopShapingController, integralGainStateController=integralGainStateController, feedbackGainStateController=feedbackGainStateController, sysMatrixAdObserver=sysMatrixAdObserver, sysMatrixBduObserver=sysMatrixBduObserver, sysMatrixCdObserver=sysMatrixCdObserver, feedbackGainObserver=feedbackGainObserver}
      mask prompts: constParam "Constant:"; controllerSel "Controller Selector:"; proportionalGainPidController "Proportional Gain PID Controller:"; integralGainPidController "Integral Gain PI Controller:"; numzTfLoopShapingController "Numerator Transfer Function Loop Shaping Controller:"; denzTfLoopShapingController "Denumerator Transfer Function Loop Shaping Controller:"; integralGainStateController "Integral Gain State Controller:"; feedbackGainStateController "Feedback Gain State Controller:"; sysMatrixAdObserver "System Matrix Ad Observer:"; sysMatrixBduObserver "System Matrix Bdu Observer:"; sysMatrixCdObserver "System Matrix Cd Observer:"; feedbackGainObserver "Feedback Gain Oberver:"
  fcnState : Outport  InitialOutput=0
  refVoltageMot1 : Outport  Port=2  InitialOutput=0.0
  refCurrentMot2 : Outport  Port=3  InitialOutput=0.0
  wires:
  Mux/1 -> To Workspace/1
  Constant3/1 -> refCurrentMot2/1
  controller/1(refVoltagMot1) -> Gain/1, Mux/1
  Unit Delay1/1 -> controlStepSequenze/3(time), Add1/2, Mux/4
  Add1/1 -> Unit Delay1/1
  Constant2/1 -> Add1/1
  controlStepSequenze/1(fcnState) -> fcnState/1
  controlStepSequenze/2(stepVal) -> Mux/3, controller/1(refVelMot1)
  Constant1/1 -> controlStepSequenze/2(stepSeq)
  Constant/1 -> controlStepSequenze/1(nrOfSteps)
  estimatedVelMot1/1 -> Mux/2, controller/2(estimatedVelMot1)
  Gain/1 -> refVoltageMot1/1

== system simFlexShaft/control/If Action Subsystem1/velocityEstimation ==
  note: delta or relative
  deltaPosMot1 : Inport
  Discrete Filter : DiscreteFilter  Numerator=constParam.lowpass.numz.*1  Denominator=constParam.lowpass.denz.*1
  Gain1 : Gain  Gain=constParam.invSamplingTime*1
  estimatedVelMot1 : Outport
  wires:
  Gain1/1 -> Discrete Filter/1
  deltaPosMot1/1 -> Gain1/1
  Discrete Filter/1 -> estimatedVelMot1/1

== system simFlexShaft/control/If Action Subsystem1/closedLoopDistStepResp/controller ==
  refVelMot1 : Inport
  estimatedVelMot1 : Inport  Port=2
  Constant : Constant  Value=controllerSel  OutDataTypeMode=uint8  OutDataTypeStr=uint8
  Merge1 : Merge  Inputs=3
  Switch Case1 : SwitchCase  CaseConditions={0,1,2}  ShowDefaultCase=off
  loopShaping : Subsystem  TreatAsAtomicUnit=on  mask{constParam=constParam.loopShaping, numz=numzTfLoopShapingController, denz=denzTfLoopShapingController}
      mask prompts: constParam "Constant:"; numz "Numerator Transfer Function Controller:"; denz "Denumerator Transfer Function Controller:"
  pid : Subsystem  TreatAsAtomicUnit=on  mask{constParam=constParam.pid, Kp=proportionalGainPidController, Ki=integralGainPidController}
      mask prompts: constParam "Constant:"; Kp "Proportional Gain Controller:"; Ki "Integral Gain Controller:"
  state : Subsystem  TreatAsAtomicUnit=on  mask{constParam=constParam.state, Ki=integralGainStateController, K=feedbackGainStateController, Ad=sysMatrixAdObserver, Bdu=sysMatrixBduObserver, Cd=sysMatrixCdObserver, L=feedbackGainObserver}
      mask prompts: constParam "Constant:"; Ki "Integral Gain State Controller:"; K "Feedback Gain State Controller:"; Ad "System Matrix Ad Oberver:"; Bdu "System Matrix Bdu Observer:"; Cd "System Matrix Cd Observer:"; L "Feedback Gain Observer:"
  refVoltagMot1 : Outport  InitialOutput=0.0
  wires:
  Switch Case1/1 -> pid/Action
  loopShaping/1(refVoltageMot1) -> Merge1/2
  state/1(refVoltageMot1) -> Merge1/3
  pid/1(refVoltageMot1) -> Merge1/1
  Switch Case1/3 -> state/Action
  Switch Case1/2 -> loopShaping/Action
  Constant/1 -> Switch Case1/1
  estimatedVelMot1/1 -> pid/2(estimatedVelMot1), loopShaping/2(estimatedVelMot1), state/2(estimatedVelMot1)
  refVelMot1/1 -> pid/1(refVelMot1), loopShaping/1(refVelMot1), state/1(refVelMot1)
  Merge1/1 -> refVoltagMot1/1

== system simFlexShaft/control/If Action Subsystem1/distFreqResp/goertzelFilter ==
  xk : Inport
  ak : Inport  Port=2
  Enable : EnablePort  StatesWhenEnabling=reset
  Add1 : Sum  Inputs=+-+
  Mux : Mux  Inputs=2
  Product : Product
  Unit Delay : UnitDelay  X0=0.0  SampleTime=-1
  Unit Delay1 : UnitDelay  X0=0.0  SampleTime=-1
  vk : Outport  InitialOutput=0
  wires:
  Unit Delay1/1 -> Unit Delay/1, Product/1, Mux/2
  Add1/1 -> Unit Delay1/1, Mux/1
  xk/1 -> Add1/1
  Product/1 -> Add1/3
  Unit Delay/1 -> Add1/2
  ak/1 -> Product/2
  Mux/1 -> vk/1

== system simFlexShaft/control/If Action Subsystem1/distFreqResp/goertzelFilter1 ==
  xk : Inport
  ak : Inport  Port=2
  Enable : EnablePort  StatesWhenEnabling=reset
  Add1 : Sum  Inputs=+-+
  Mux : Mux  Inputs=2
  Product : Product
  Unit Delay : UnitDelay  X0=0.0  SampleTime=-1
  Unit Delay1 : UnitDelay  X0=0.0  SampleTime=-1
  vk : Outport  InitialOutput=0
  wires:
  Unit Delay1/1 -> Unit Delay/1, Product/1, Mux/2
  Add1/1 -> Unit Delay1/1, Mux/1
  xk/1 -> Add1/1
  Product/1 -> Add1/3
  Unit Delay/1 -> Add1/2
  ak/1 -> Product/2
  Mux/1 -> vk/1

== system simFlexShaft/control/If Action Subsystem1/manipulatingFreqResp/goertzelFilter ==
  xk : Inport
  ak : Inport  Port=2
  Enable : EnablePort  StatesWhenEnabling=reset
  Add1 : Sum  Inputs=+-+
  Mux : Mux  Inputs=2
  Product : Product
  Unit Delay : UnitDelay  X0=0.0  SampleTime=-1
  Unit Delay1 : UnitDelay  X0=0.0  SampleTime=-1
  vk : Outport  InitialOutput=0
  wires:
  Unit Delay1/1 -> Unit Delay/1, Product/1, Mux/2
  Add1/1 -> Unit Delay1/1, Mux/1
  xk/1 -> Add1/1
  Product/1 -> Add1/3
  Unit Delay/1 -> Add1/2
  ak/1 -> Product/2
  Mux/1 -> vk/1

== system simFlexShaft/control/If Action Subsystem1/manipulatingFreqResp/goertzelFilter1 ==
  xk : Inport
  ak : Inport  Port=2
  Enable : EnablePort  StatesWhenEnabling=reset
  Add1 : Sum  Inputs=+-+
  Mux : Mux  Inputs=2
  Product : Product
  Unit Delay : UnitDelay  X0=0.0  SampleTime=-1
  Unit Delay1 : UnitDelay  X0=0.0  SampleTime=-1
  vk : Outport  InitialOutput=0
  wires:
  Unit Delay1/1 -> Unit Delay/1, Product/1, Mux/2
  Add1/1 -> Unit Delay1/1, Mux/1
  xk/1 -> Add1/1
  Product/1 -> Add1/3
  Unit Delay/1 -> Add1/2
  ak/1 -> Product/2
  Mux/1 -> vk/1

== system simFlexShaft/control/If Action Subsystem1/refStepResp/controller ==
  refVelMot1 : Inport
  estimatedVelMot1 : Inport  Port=2
  Constant : Constant  Value=controllerSel  OutDataTypeMode=uint8  OutDataTypeStr=uint8
  Merge1 : Merge  Inputs=3
  Switch Case1 : SwitchCase  CaseConditions={0,1,2}  ShowDefaultCase=off
  loopShaping : Subsystem  TreatAsAtomicUnit=on  mask{constParam=constParam.loopShaping, numz=numzTfLoopShapingController, denz=denzTfLoopShapingController}
      mask prompts: constParam "Constant:"; numz "Numerator Transfer Function Controller:"; denz "Denumerator Transfer Function Controller:"
  pid : Subsystem  TreatAsAtomicUnit=on  mask{constParam=constParam.pid, Kp=proportionalGainPidController, Ki=integralGainPidController}
      mask prompts: constParam "Constant:"; Kp "Proportional Gain Controller:"; Ki "Integral Gain Controller:"
  state : Subsystem  TreatAsAtomicUnit=on  mask{constParam=constParam.state, Ki=integralGainStateController, K=feedbackGainStateController, Ad=sysMatrixAdObserver, Bdu=sysMatrixBduObserver, Cd=sysMatrixCdObserver, L=feedbackGainObserver}
      mask prompts: constParam "Constant:"; Ki "Integral Gain State Controller:"; K "Feedback Gain State Controller:"; Ad "System Matrix Ad Oberver:"; Bdu "System Matrix Bdu Observer:"; Cd "System Matrix Cd Observer:"; L "Feedback Gain Observer:"
  refVoltagMot1 : Outport  InitialOutput=0.0
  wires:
  Switch Case1/1 -> pid/Action
  loopShaping/1(refVoltageMot1) -> Merge1/2
  state/1(refVoltageMot1) -> Merge1/3
  pid/1(refVoltageMot1) -> Merge1/1
  Switch Case1/3 -> state/Action
  Switch Case1/2 -> loopShaping/Action
  Constant/1 -> Switch Case1/1
  estimatedVelMot1/1 -> pid/2(estimatedVelMot1), loopShaping/2(estimatedVelMot1), state/2(estimatedVelMot1)
  refVelMot1/1 -> pid/1(refVelMot1), loopShaping/1(refVelMot1), state/1(refVelMot1)
  Merge1/1 -> refVoltagMot1/1

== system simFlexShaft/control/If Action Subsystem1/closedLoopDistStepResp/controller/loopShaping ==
  refVelMot1 : Inport
  estimatedVelMot1 : Inport  Port=2
  Action Port : ActionPort  InitializeStates=reset  ActionType=case
  Discrete Transfer Fcn : DiscreteTransferFcn  Numerator=numz  Denominator=denz  SampleTime=-1
  Saturation : Saturate  UpperLimit=constParam.refVoltageLimMot1  LowerLimit=-constParam.refVoltageLimMot1
  Subtract1 : Sum  Inputs=+-
  refVoltageMot1 : Outport  InitialOutput=0.0
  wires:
  refVelMot1/1 -> Subtract1/1
  estimatedVelMot1/1 -> Subtract1/2
  Subtract1/1 -> Discrete Transfer Fcn/1
  Discrete Transfer Fcn/1 -> Saturation/1
  Saturation/1 -> refVoltageMot1/1

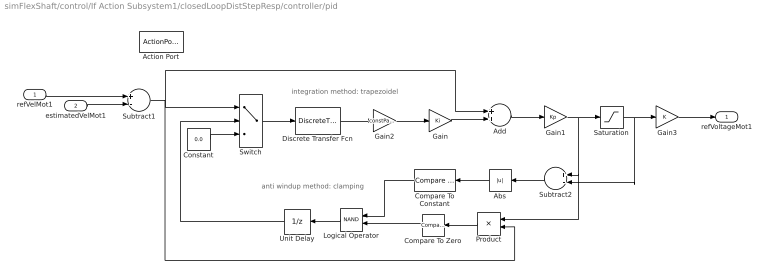
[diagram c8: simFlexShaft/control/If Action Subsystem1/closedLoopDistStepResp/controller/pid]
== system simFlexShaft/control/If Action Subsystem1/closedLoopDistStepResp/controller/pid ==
  note: integration method: trapezoidel
  note: anti windup method: clamping
  refVelMot1 : Inport
  estimatedVelMot1 : Inport  Port=2
  Action Port : ActionPort  InitializeStates=reset  ActionType=case
  Abs : Abs
  Add : Sum
  Compare To Constant : simulink/Logic and Bit Operations/Compare To Constant  SystemSampleTime=-1  relop=>  const=1e-3  LogicOutDataTypeMode=uint8
  Compare To Zero : simulink/Logic and Bit Operations/Compare To Zero  SystemSampleTime=-1  relop=>  LogicOutDataTypeMode=uint8
  Constant : Constant  Value=0.0
  Discrete Transfer Fcn : DiscreteTransferFcn  Numerator=[1 1]  Denominator=[1 -1]  SampleTime=-1
  Gain : Gain  Gain=Ki
  Gain1 : Gain  Gain=Kp
  Gain2 : Gain  Gain=constParam.halfSamplingTime
  Gain3 : Gain
  Logical Operator : Logic  Operator=NAND  AllPortsSameDT=off  OutDataTypeMode=boolean  OutDataTypeStr=boolean
  Product : Product
  Saturation : Saturate  UpperLimit=constParam.refVoltageLimMot1  LowerLimit=-constParam.refVoltageLimMot1
  Subtract1 : Sum  Inputs=+-
  Subtract2 : Sum  Inputs=+-
  Switch : Switch  Criteria=u2 > Threshold
  Unit Delay : UnitDelay  SampleTime=-1
  refVoltageMot1 : Outport  InitialOutput=0.0
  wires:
  refVelMot1/1 -> Subtract1/1
  estimatedVelMot1/1 -> Subtract1/2
  Discrete Transfer Fcn/1 -> Gain2/1
  Gain/1 -> Add/2
  Gain1/1 -> Saturation/1, Product/1, Subtract2/1
  Subtract1/1 -> Add/1, Switch/1, Product/2
  Gain2/1 -> Gain/1
  Add/1 -> Gain1/1
  Switch/1 -> Discrete Transfer Fcn/1
  Constant/1 -> Switch/3
  Saturation/1 -> Gain3/1, Subtract2/2
  Logical Operator/1 -> Unit Delay/1
  Unit Delay/1 -> Switch/2
  Compare To Zero/1 -> Logical Operator/2
  Gain3/1 -> refVoltageMot1/1
  Subtract2/1 -> Abs/1
  Abs/1 -> Compare To Constant/1
  Product/1 -> Compare To Zero/1
  Compare To Constant/1 -> Logical Operator/1

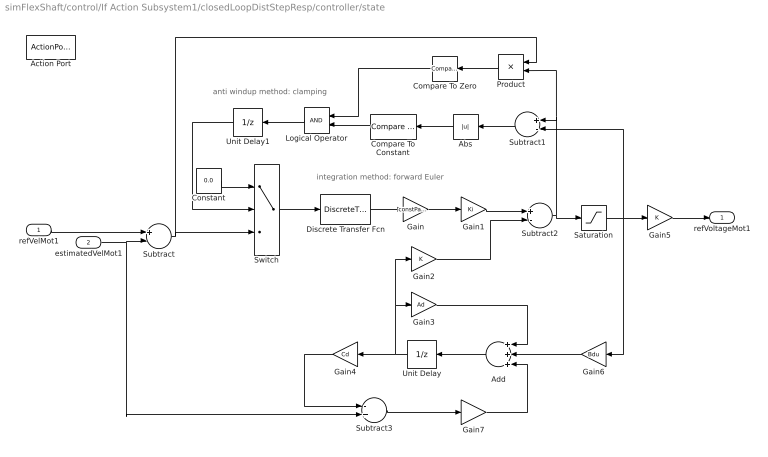
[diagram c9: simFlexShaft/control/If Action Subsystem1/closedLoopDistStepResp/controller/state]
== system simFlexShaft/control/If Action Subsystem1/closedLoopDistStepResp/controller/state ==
  note: anti windup method: clamping
  note: integration method: forward Euler
  refVelMot1 : Inport
  estimatedVelMot1 : Inport  Port=2
  Action Port : ActionPort  InitializeStates=reset  ActionType=case
  Abs : Abs
  Add : Sum  Inputs=+++
  Compare To Constant : simulink/Logic and Bit Operations/Compare To Constant  SystemSampleTime=-1  relop=>  const=1e-3  LogicOutDataTypeMode=uint8
  Compare To Zero : simulink/Logic and Bit Operations/Compare To Zero  SystemSampleTime=-1  relop=>  LogicOutDataTypeMode=uint8
  Constant : Constant  Value=0.0
  Discrete Transfer Fcn : DiscreteTransferFcn  Denominator=[1 -1]  SampleTime=-1
  Gain : Gain  Gain=constParam.samplingTime
  Gain1 : Gain  Gain=Ki
  Gain2 : Gain  Gain=K  Multiplication=Matrix(K*u)
  Gain3 : Gain  Gain=Ad  Multiplication=Matrix(K*u)
  Gain4 : Gain  Gain=Cd  Multiplication=Matrix(K*u)
  Gain5 : Gain
  Gain6 : Gain  Gain=Bdu  Multiplication=Matrix(K*u)
  Gain7 : Gain  Gain=L  Multiplication=Matrix(K*u)
  Logical Operator : Logic  AllPortsSameDT=off  OutDataTypeMode=boolean  OutDataTypeStr=boolean
  Product : Product
  Saturation : Saturate  UpperLimit=constParam.refVoltageLimMot1  LowerLimit=-constParam.refVoltageLimMot1
  Subtract : Sum  Inputs=+-
  Subtract1 : Sum  Inputs=+-
  Subtract2 : Sum  Inputs=+-
  Subtract3 : Sum  Inputs=-+
  Switch : Switch  Criteria=u2 > Threshold
  Unit Delay : UnitDelay  SampleTime=-1
  Unit Delay1 : UnitDelay  SampleTime=-1
  refVoltageMot1 : Outport  InitialOutput=0.0
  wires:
  Subtract2/1 -> Saturation/1, Product/2, Subtract1/1
  Gain6/1 -> Add/2
  Add/1 -> Unit Delay/1
  Unit Delay/1 -> Gain4/1, Gain3/1, Gain2/1
  refVelMot1/1 -> Subtract/1
  estimatedVelMot1/1 -> Subtract/2, Subtract3/2
  Gain3/1 -> Add/1
  Gain4/1 -> Subtract3/1
  Discrete Transfer Fcn/1 -> Gain/1
  Gain5/1 -> refVoltageMot1/1
  Saturation/1 -> Gain6/1, Gain5/1, Subtract1/2
  Subtract3/1 -> Gain7/1
  Gain7/1 -> Add/3
  Gain/1 -> Gain1/1
  Gain1/1 -> Subtract2/1
  Gain2/1 -> Subtract2/2
  Product/1 -> Compare To Zero/1
  Logical Operator/1 -> Unit Delay1/1
  Compare To Constant/1 -> Logical Operator/2
  Compare To Zero/1 -> Logical Operator/1
  Unit Delay1/1 -> Switch/2
  Subtract/1 -> Switch/3, Product/1
  Constant/1 -> Switch/1
  Switch/1 -> Discrete Transfer Fcn/1
  Subtract1/1 -> Abs/1
  Abs/1 -> Compare To Constant/1

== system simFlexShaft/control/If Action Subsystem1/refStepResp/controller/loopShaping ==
  refVelMot1 : Inport
  estimatedVelMot1 : Inport  Port=2
  Action Port : ActionPort  InitializeStates=reset  ActionType=case
  Discrete Transfer Fcn : DiscreteTransferFcn  Numerator=numz  Denominator=denz  SampleTime=-1
  Saturation : Saturate  UpperLimit=constParam.refVoltageLimMot1  LowerLimit=-constParam.refVoltageLimMot1
  Subtract1 : Sum  Inputs=+-
  refVoltageMot1 : Outport  InitialOutput=0.0
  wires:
  refVelMot1/1 -> Subtract1/1
  estimatedVelMot1/1 -> Subtract1/2
  Subtract1/1 -> Discrete Transfer Fcn/1
  Discrete Transfer Fcn/1 -> Saturation/1
  Saturation/1 -> refVoltageMot1/1

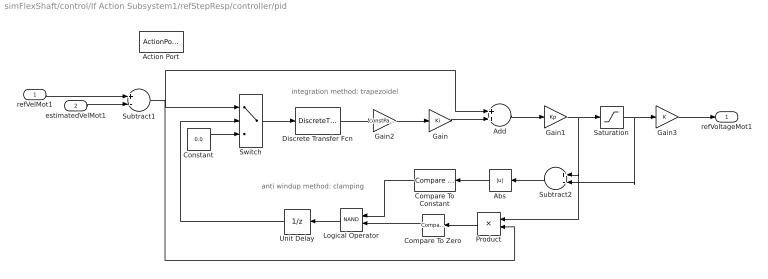
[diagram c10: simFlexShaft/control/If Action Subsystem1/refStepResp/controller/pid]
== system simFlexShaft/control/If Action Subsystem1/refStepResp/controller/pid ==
  note: integration method: trapezoidel
  note: anti windup method: clamping
  refVelMot1 : Inport
  estimatedVelMot1 : Inport  Port=2
  Action Port : ActionPort  InitializeStates=reset  ActionType=case
  Abs : Abs
  Add : Sum
  Compare To Constant : simulink/Logic and Bit Operations/Compare To Constant  SystemSampleTime=-1  relop=>  const=1e-3  LogicOutDataTypeMode=uint8
  Compare To Zero : simulink/Logic and Bit Operations/Compare To Zero  SystemSampleTime=-1  relop=>  LogicOutDataTypeMode=uint8
  Constant : Constant  Value=0.0
  Discrete Transfer Fcn : DiscreteTransferFcn  Numerator=[1 1]  Denominator=[1 -1]  SampleTime=-1
  Gain : Gain  Gain=Ki
  Gain1 : Gain  Gain=Kp
  Gain2 : Gain  Gain=constParam.halfSamplingTime
  Gain3 : Gain
  Logical Operator : Logic  Operator=NAND  AllPortsSameDT=off  OutDataTypeMode=boolean  OutDataTypeStr=boolean
  Product : Product
  Saturation : Saturate  UpperLimit=constParam.refVoltageLimMot1  LowerLimit=-constParam.refVoltageLimMot1
  Subtract1 : Sum  Inputs=+-
  Subtract2 : Sum  Inputs=+-
  Switch : Switch  Criteria=u2 > Threshold
  Unit Delay : UnitDelay  SampleTime=-1
  refVoltageMot1 : Outport  InitialOutput=0.0
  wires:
  refVelMot1/1 -> Subtract1/1
  estimatedVelMot1/1 -> Subtract1/2
  Discrete Transfer Fcn/1 -> Gain2/1
  Gain/1 -> Add/2
  Gain1/1 -> Saturation/1, Product/1, Subtract2/1
  Subtract1/1 -> Add/1, Switch/1, Product/2
  Gain2/1 -> Gain/1
  Add/1 -> Gain1/1
  Switch/1 -> Discrete Transfer Fcn/1
  Constant/1 -> Switch/3
  Saturation/1 -> Gain3/1, Subtract2/2
  Logical Operator/1 -> Unit Delay/1
  Unit Delay/1 -> Switch/2
  Compare To Zero/1 -> Logical Operator/2
  Gain3/1 -> refVoltageMot1/1
  Subtract2/1 -> Abs/1
  Abs/1 -> Compare To Constant/1
  Product/1 -> Compare To Zero/1
  Compare To Constant/1 -> Logical Operator/1

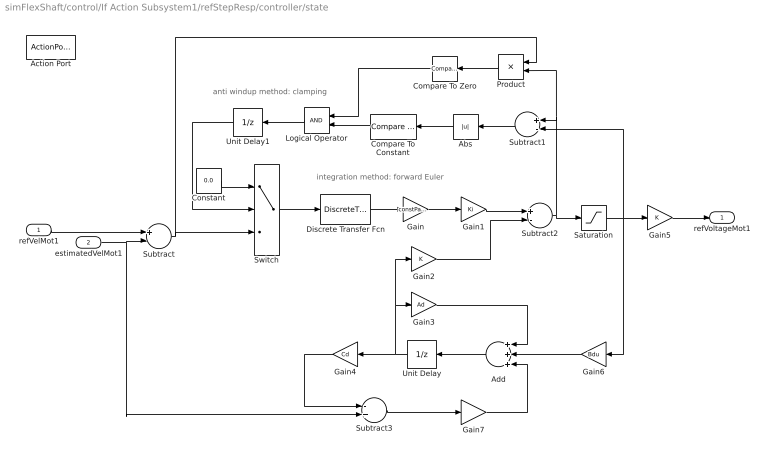
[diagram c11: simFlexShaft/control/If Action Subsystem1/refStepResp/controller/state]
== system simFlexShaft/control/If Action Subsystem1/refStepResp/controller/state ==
  note: anti windup method: clamping
  note: integration method: forward Euler
  refVelMot1 : Inport
  estimatedVelMot1 : Inport  Port=2
  Action Port : ActionPort  InitializeStates=reset  ActionType=case
  Abs : Abs
  Add : Sum  Inputs=+++
  Compare To Constant : simulink/Logic and Bit Operations/Compare To Constant  SystemSampleTime=-1  relop=>  const=1e-3  LogicOutDataTypeMode=uint8
  Compare To Zero : simulink/Logic and Bit Operations/Compare To Zero  SystemSampleTime=-1  relop=>  LogicOutDataTypeMode=uint8
  Constant : Constant  Value=0.0
  Discrete Transfer Fcn : DiscreteTransferFcn  Denominator=[1 -1]  SampleTime=-1
  Gain : Gain  Gain=constParam.samplingTime
  Gain1 : Gain  Gain=Ki
  Gain2 : Gain  Gain=K  Multiplication=Matrix(K*u)
  Gain3 : Gain  Gain=Ad  Multiplication=Matrix(K*u)
  Gain4 : Gain  Gain=Cd  Multiplication=Matrix(K*u)
  Gain5 : Gain
  Gain6 : Gain  Gain=Bdu  Multiplication=Matrix(K*u)
  Gain7 : Gain  Gain=L  Multiplication=Matrix(K*u)
  Logical Operator : Logic  AllPortsSameDT=off  OutDataTypeMode=boolean  OutDataTypeStr=boolean
  Product : Product
  Saturation : Saturate  UpperLimit=constParam.refVoltageLimMot1  LowerLimit=-constParam.refVoltageLimMot1
  Subtract : Sum  Inputs=+-
  Subtract1 : Sum  Inputs=+-
  Subtract2 : Sum  Inputs=+-
  Subtract3 : Sum  Inputs=-+
  Switch : Switch  Criteria=u2 > Threshold
  Unit Delay : UnitDelay  SampleTime=-1
  Unit Delay1 : UnitDelay  SampleTime=-1
  refVoltageMot1 : Outport  InitialOutput=0.0
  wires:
  Subtract2/1 -> Saturation/1, Product/2, Subtract1/1
  Gain6/1 -> Add/2
  Add/1 -> Unit Delay/1
  Unit Delay/1 -> Gain4/1, Gain3/1, Gain2/1
  refVelMot1/1 -> Subtract/1
  estimatedVelMot1/1 -> Subtract/2, Subtract3/2
  Gain3/1 -> Add/1
  Gain4/1 -> Subtract3/1
  Discrete Transfer Fcn/1 -> Gain/1
  Gain5/1 -> refVoltageMot1/1
  Saturation/1 -> Gain6/1, Gain5/1, Subtract1/2
  Subtract3/1 -> Gain7/1
  Gain7/1 -> Add/3
  Gain/1 -> Gain1/1
  Gain1/1 -> Subtract2/1
  Gain2/1 -> Subtract2/2
  Product/1 -> Compare To Zero/1
  Logical Operator/1 -> Unit Delay1/1
  Compare To Constant/1 -> Logical Operator/2
  Compare To Zero/1 -> Logical Operator/1
  Unit Delay1/1 -> Switch/2
  Subtract/1 -> Switch/3, Product/1
  Constant/1 -> Switch/1
  Switch/1 -> Discrete Transfer Fcn/1
  Subtract1/1 -> Abs/1
  Abs/1 -> Compare To Constant/1
